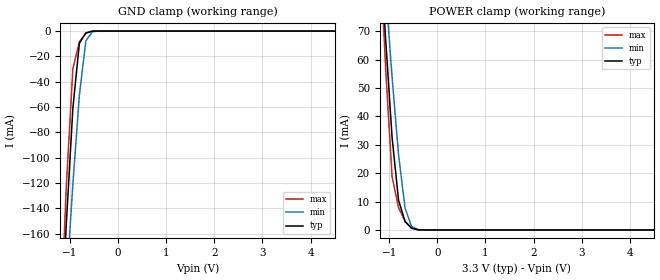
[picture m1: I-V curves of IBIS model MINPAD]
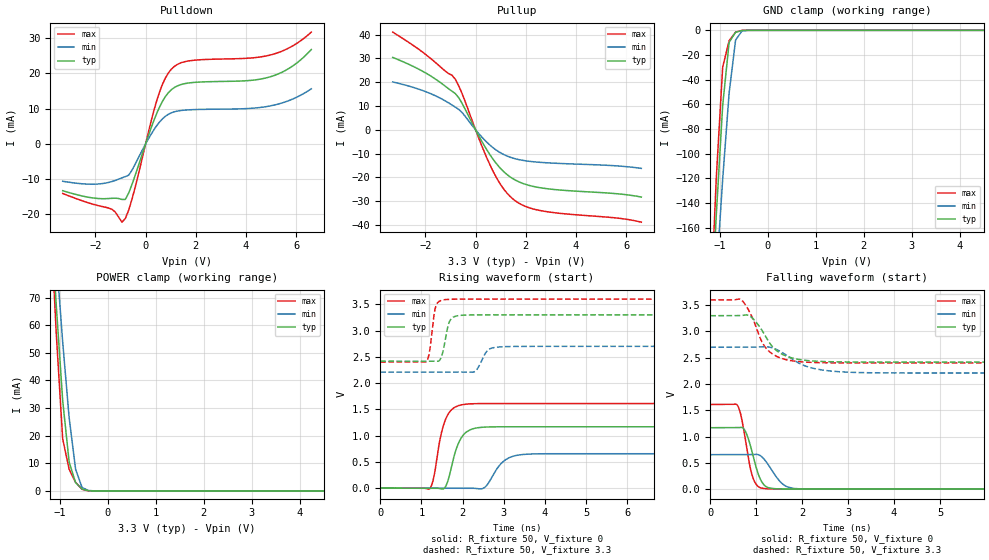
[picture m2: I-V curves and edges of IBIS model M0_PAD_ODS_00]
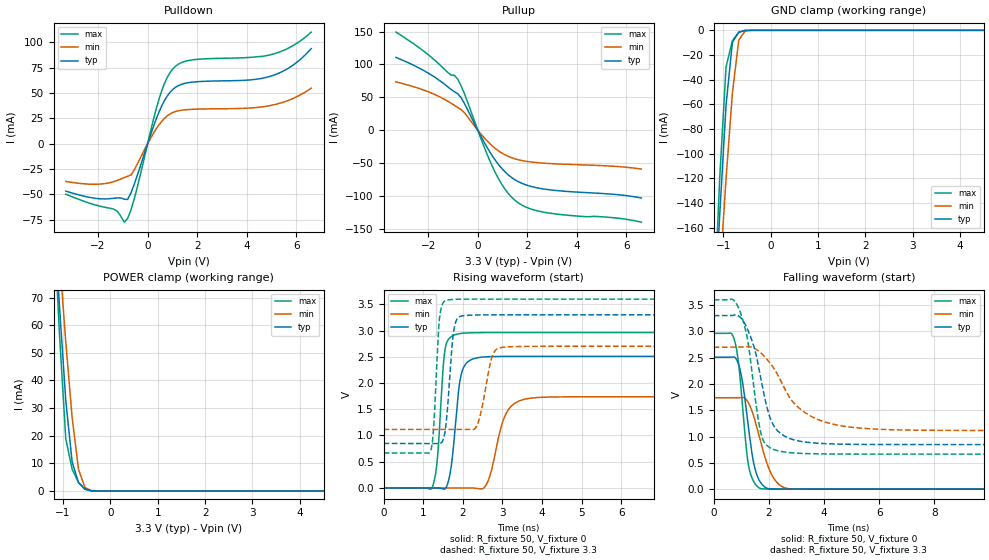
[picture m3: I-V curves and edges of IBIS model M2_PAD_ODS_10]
|   Microsemi Corporation
|   SmartFusion2 Automotive IBIS Model
[IBIS ver]   5.0
[File name]   as30208cc_33v_rev2p11.ibs
[File Rev]   2.11
[Date]   Wed Jul 17 2024
[Source] Simulated Models ONLY.
   All data is based on Spice simulation. All performed at Microsemi Corporation.
   Please refer to the Microsemi website for future updates at www.microsemi.com
[Notes]  Microsemi SmartFusion2 IBIS models for automotive operating conditions
   for DDRIO IO Banks IO Configurations ONLY. Models uses a software default
   fixed codes except for DDR3/SSTL15 which will always require calibrated
   codes.
   Automotive Temperature Grade 2 (t2) models cover a temperature range from
   -40C to 125C.
   Please refer to msio_auto_t2.ibs for MSIO IO Banks IO Configurations.
   Please refer to msiod_auto_t2.ibs for MSIOD IO Banks IO Configurations.
   The package parasitics of various package types are given.
   Uncomment the appropriate package or refer to the .pkg for specific
   per pin parasitic data.
   There are warnings related to non-monotonic and Increasing/Decreasing Current.
   They are expected on 20 Ohms and 30 Ohms I/O ODT models in DDR3/SSTL15.
[Disclaimer] This information is for board design considerations.
   Simulation based V/I curves contained in this model file are
   considered preliminary until verified against bench
   measurements. Maximum currents may vary from part to part but
   should not exceed maximum I/V curves provided in this model file.
[Copyright]  (c) 2015, Microsemi Corporation, All Rights Reserved.
| IBIS MODEL CHECKLIST
| Microsemi is dedicated to releasing quality IBIS models to customers.
| The following items have been
| verified for this IBIS model before release:
| 1)  Checked IBIS model by the golden parser ibischk5 [Complete]
| 2)  Ensured no errors reported by golden parser
|   for the IBIS model [Complete]
| 3)  Defined Vinl and Vinh for recievers [Complete]
| 4)  Defined Standard Load and Vmeas values for drivers [Complete]
| 5)  Defined overshoots for drivers and recievers [NA]
| 6)  Validated Ramp Values[Complete]
| 7)  Defined V-T Tables for all output drivers [Complete]
| 8)  Validated [Diff Pins] []
| 9)  Verified Package Parasitics [Complete]
| 10) Defined Standard Load Parameters and Specifications
|   for waveforms [Complete]
| 11) Defined and Validate Pin mappings [Complete]
| 12) Verified Ccomp Value []
| 13) Visually Inspected I-V Curves and V-T Tables  [Complete]
| 14) Presented Typ/Min/Max Values in the correct order for
|   all tables and parameters [Complete]
| 15) Simulated all output models with standard load and
|   switching through Vmeas [Complete]
| 16) Simulated all reciever models  [Complete]
| 17) Validated Models selectors. []
| 18) Visually inspected Spice and IBIS correlation for
|   a) Typical VT Curves [Complete]
|   b) Minimum VT Curves [Complete]
|   c) Maximum VT Curves [Complete]
| 19) Visually inspected Silicon and IBIS correlation
|   a) Typical IV Pull UP/ Pull Down Curves []
|   b) Minimum IV Pull UP/ Pull Down Curves []
|   c) Maximum IV Pull UP/ Pull Down Curves []
|   Component SmartFusion2
[Component]   SmartFusion2 W MRAM
[Manufacturer]   Avalanche Technology
[Package]
|  Design die-package: BGA
| variable   typ   min   max
R_pkg   0.72029   0.51528   1.0002
L_pkg   5.797e-9   4.155e-9   8.073e-9
C_pkg   1.116e-12   7.907e-13   1.753e-12
|Pin and Model info
[Pin]  signal_name  model_name   R_pin   L_pin   C_pin
L7   CS1#   MINPAD   0.4340		15.2000E-9		1.2600E-12
J8   CS2#   MINPAD   0.3800		13.5000E-9		1.0400E-12
K7   CLK1   MINPAD   0.4300		12.7000E-9		0.9790E-12
K6   CLK2   MINPAD   0.4480		14.6000E-9		1.1600E-12
M8   IO_0   MIOPAD   0.4010		12.4000E-9		1.2500E-12
M7   IO_1   MIOPAD   0.4050		14.2000E-9		1.1100E-12
L9   IO_2   MIOPAD   0.3780		11.8000E-9		1.2000E-12
M9   IO_3   MIOPAD   0.3700		11.8000E-9		1.2600E-12
M10   IO_4   MIOPAD   0.3710		11.1000E-9		1.1000E-12
N8   IO_5   MIOPAD   0.4050		13.8000E-9		1.1600E-12
N7   IO_6   MIOPAD   0.3830		15.2000E-9		1.0900E-12
N6   IO_7   MIOPAD   0.4480		16.4000E-9		1.0800E-12
J12   HTBSEL   MINPAD   0.1380		6.1700E-9		0.6060E-12
H12   HBP_2   MINPAD   0.1470		6.3900E-9		1.0000E-12
G11   HBP_1   MINPAD   0.1910		8.5000E-9		1.1500E-12
G10   HBP_0   MINPAD   0.2050		8.6800E-9		1.4200E-12
J9   RESET#   MINPAD   0.3410		14.1000E-9		1.6300E-12
J10   INT1#   MIOPAD   0.3080		12.5000E-9		1.2100E-12
K8   INT2#   MIOPAD   0.2120		10.3000E-9		0.8230E-12
M5   VSSIO   GND   NA   NA   NA
H6   VSSIO   GND   NA   NA   NA
L6   VSSIO   GND   NA   NA   NA
P8   VSSIO   GND   NA   NA   NA
H10   VSSIO   GND   NA   NA   NA
N10   VSSIO   GND   NA   NA   NA
P10   VSSIO   GND   NA   NA   NA
H11   VSSIO   GND   NA   NA   NA
N11   VSSIO   GND   NA   NA   NA
A1   VSS   GND   NA   NA   NA
B1   VSS   GND   NA   NA   NA
W1   VSS   GND   NA   NA   NA
Y1   VSS   GND   NA   NA   NA
A2   VSS   GND   NA   NA   NA
Y2   VSS   GND   NA   NA   NA
F3   VSS   GND   NA   NA   NA
G3   VSS   GND   NA   NA   NA
P3   VSS   GND   NA   NA   NA
R3   VSS   GND   NA   NA   NA
F4   VSS   GND   NA   NA   NA
H4   VSS   GND   NA   NA   NA
J4   VSS   GND   NA   NA   NA
L4   VSS   GND   NA   NA   NA
N4   VSS   GND   NA   NA   NA
R4   VSS   GND   NA   NA   NA
L5   VSS   GND   NA   NA   NA
N5   VSS   GND   NA   NA   NA
G6   VSS   GND   NA   NA   NA
P6   VSS   GND   NA   NA   NA
G8   VSS   GND   NA   NA   NA
H8   VSS   GND   NA   NA   NA
L10   VSS   GND   NA   NA   NA
L11   VSS   GND   NA   NA   NA
P11   VSS   GND   NA   NA   NA
F12   VSS   GND   NA   NA   NA
L12   VSS   GND   NA   NA   NA
N12   VSS   GND   NA   NA   NA
R12   VSS   GND   NA   NA   NA
F13   VSS   GND   NA   NA   NA
G13   VSS   GND   NA   NA   NA
P13   VSS   GND   NA   NA   NA
R13   VSS   GND   NA   NA   NA
A14   VSS   GND   NA   NA   NA
Y14   VSS   GND   NA   NA   NA
A15   VSS   GND   NA   NA   NA
B15   VSS   GND   NA   NA   NA
W15   VSS   GND   NA   NA   NA
Y15   VSS   GND   NA   NA   NA
G4   VCCIO   POWER   NA   NA   NA
P4   VCCIO   POWER   NA   NA   NA
G5   VCCIO   POWER   NA   NA   NA
J5   VCCIO   POWER   NA   NA   NA
P5   VCCIO   POWER   NA   NA   NA
M6   VCCIO   POWER   NA   NA   NA
H7   VCCIO   POWER   NA   NA   NA
H9   VCCIO   POWER   NA   NA   NA
N9   VCCIO   POWER   NA   NA   NA
J11   VCCIO   POWER   NA   NA   NA
M11   VCCIO   POWER   NA   NA   NA
G12   VCCIO   POWER   NA   NA   NA
P12   VCCIO   POWER   NA   NA   NA
K4   VCC   POWER   NA   NA   NA
M4   VCC   POWER   NA   NA   NA
K5   VCC   POWER   NA   NA   NA
G7   VCC   POWER   NA   NA   NA
P7   VCC   POWER   NA   NA   NA
G9   VCC   POWER   NA   NA   NA
K9   VCC   POWER   NA   NA   NA
P9   VCC   POWER   NA   NA   NA
K11   VCC   POWER   NA   NA   NA
K12   VCC   POWER   NA   NA   NA
M12   VCC   POWER   NA   NA   NA
| END PIN INFO
| IOPAD
[Model Selector] MIOPAD
| Model Description
M0_PAD_ODS_00   ODS_00
M1_PAD_ODS_01   ODS_01
M2_PAD_ODS_10   ODS_10
M3_PAD_ODS_11   ODS_11
| Models and submodels in the file (5): MINPAD (Input), M0_PAD_ODS_00 (I/O), M2_PAD_ODS_10 (I/O), M1_PAD_ODS_01 (I/O), M3_PAD_ODS_11 (I/O)
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[Model] MINPAD
Model_type Input
Enable   Active-High
Vinl  =  0.8
Vinh  =  2.2
| Capacitance  typ   min   max
C_comp   1.514821e-12   1.418868e-12   1.647023e-12
| Variables   typ   min   max
[GND Clamp Reference]   0   0   0
[POWER Clamp Reference]   3.3   2.7   3.6
[Pulldown Reference]   0   0   0
[Pullup Reference]   3.3   2.7   3.6
[Temperature Range]   25   125   -40
[Voltage Range]   3.3   2.7   3.6
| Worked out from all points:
|   GND clamp passes 1 mA (typ) near -0.62 V on its own axis
|   POWER clamp passes 1 mA (typ) near -0.56 V on its own axis
[GND Clamp]
| Voltage   I(typ)   I(min)   I(max)
-3.3V     -1.961A    -1.697A    -2.357A
-1.21V    -250.7mA   -283.7mA   -242.5mA
-1.076V   -150.6mA   -200.1mA   -120.6mA
-941.4mV  -60.83mA   -120.8mA   -29.75mA
-806.9mV  -9.646mA   -50.71mA   -8.435mA
-672.4mV  -1.585mA   -7.866mA   -1.457mA
-537.9mV  -71.75uA   -504.3uA   -18.73uA
-403.4mV  -593.9nA   -18.57uA   -37.22nA
6.6V      0A         0A         0A
[POWER Clamp]
| Voltage   I(typ)   I(min)   I(max)
-3.3V     772.3mA    673.3mA    930.5mA
-1.21V    105.9mA    117.6mA    104.6mA
-1.076V   67.34mA    85.06mA    57.16mA
-941.4mV  32.71mA    53.93mA    18.82mA
-806.9mV  10.48mA    26.53mA    7.848mA
-672.4mV  2.975mA    7.856mA    3.108mA
-537.9mV  710.9uA    1.248mA    573.1uA
-403.4mV  60.69uA    160.8uA    9.187uA
-269mV    142.4nA    6.118uA    23.26nA
6.6V      0A         0A         0A
[Model] M0_PAD_ODS_00
Model_type I/O
Enable   Active-High
Vinl  =  0.8
Vinh  =  2.2
Vmeas =  1.65
Cref  =  30e-12
| Capacitance  typ   min   max
C_comp   1.518749e-12   1.424706e-12   1.652746e-12
| Variables   typ   min   max
[GND Clamp Reference]   0   0   0
[POWER Clamp Reference]   3.3   2.7   3.6
[Pulldown Reference]   0   0   0
[Pullup Reference]   3.3   2.7   3.6
[Temperature Range]   25   125   -40
[Voltage Range]   3.3   2.7   3.6
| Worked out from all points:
|   slope of the pulldown table from 0 to 0.495 V, typ, clamps not added: 52.1 ohm
|   slope of the pullup table from 0 to 0.495 V, typ, clamps not added: 53.8 ohm
|   GND clamp passes 1 mA (typ) near -0.62 V on its own axis
|   POWER clamp passes 1 mA (typ) near -0.56 V on its own axis
|   falling waveform, R_fixture 50, V_fixture 0: 20-80 % time 230ps typ, 320ps min, 198ps max; typ from 1.17 V to 0 V
|   falling waveform, R_fixture 50, V_fixture 3.3: 20-80 % time 464ps typ, 644ps min, 396ps max; typ from 3.3 V to 2.42 V
|   rising waveform, R_fixture 50, V_fixture 0: 20-80 % time 273ps typ, 362ps min, 248ps max; typ from 0 V to 1.17 V
|   rising waveform, R_fixture 50, V_fixture 3.3: 20-80 % time 138ps typ, 198ps min, 114ps max; typ from 2.42 V to 3.3 V
[GND Clamp]
| Voltage   I(typ)   I(min)   I(max)
-3.3V     -1.961A    -1.697A    -2.357A
-1.21V    -250.7mA   -283.7mA   -242.5mA
-1.076V   -150.6mA   -200.1mA   -120.7mA
-941.4mV  -60.83mA   -120.8mA   -29.76mA
-806.9mV  -9.649mA   -50.71mA   -8.442mA
-672.4mV  -1.587mA   -7.866mA   -1.46mA
-537.9mV  -71.93uA   -504.3uA   -18.83uA
-403.4mV  -595.6nA   -18.58uA   -37.45nA
6.6V      0A         0A         0A
[POWER Clamp]
| Voltage   I(typ)   I(min)   I(max)
-3.3V     772.3mA    673.3mA    930.5mA
-1.21V    105.9mA    117.6mA    104.6mA
-1.076V   67.34mA    85.06mA    57.16mA
-941.4mV  32.71mA    53.93mA    18.82mA
-806.9mV  10.48mA    26.53mA    7.848mA
-672.4mV  2.975mA    7.856mA    3.108mA
-537.9mV  710.9uA    1.248mA    573.1uA
-403.4mV  60.69uA    160.8uA    9.187uA
-269mV    142.4nA    6.118uA    23.26nA
6.6V      0A         0A         0A
[Pulldown]
| Voltage   I(typ)   I(min)   I(max)
-3.3V     -13.26mA   -10.58mA   -14.05mA
-1.345V   -15.42mA   -10.67mA   -18.51mA
-941.4mV  -15.74mA   -9.611mA   -22.19mA
-806.9mV  -15.73mA   -9.263mA   -21.14mA
-537.9mV  -11.42mA   -7.417mA   -15.59mA
455.2mV   8.881mA    5.308mA    12.55mA
682.8mV   12.23mA    7.205mA    17.1mA
1.024V    15.38mA    8.837mA    21.2mA
1.821V    17.39mA    9.724mA    23.68mA
4.914V    18.96mA    10.73mA    25.16mA
5.783V    21.77mA    12.53mA    27.53mA
6.6V      26.8mA     15.66mA    31.75mA
[Pullup]
| Voltage   I(typ)   I(min)   I(max)
-3.3V     30.44mA    20.14mA    41.1mA
-1.883V   23.26mA    15.61mA    30.81mA
-806.9mV  15.23mA    9.539mA    21.27mA
-537.9mV  11.14mA    7.294mA    15.26mA
227.6mV   -4.448mA   -2.796mA   -6.209mA
682.8mV   -12.17mA   -7.42mA    -17.15mA
1.138V    -17.78mA   -10.49mA   -25.16mA
1.593V    -21.21mA   -12.21mA   -29.96mA
2.048V    -23.14mA   -13.13mA   -32.47mA
2.731V    -24.61mA   -13.8mA    -34.27mA
5.659V    -26.92mA   -15.2mA    -37.16mA
6.6V      -28.29mA   -16.23mA   -38.86mA
[Ramp]
dV/dt_r   0.701574/0.273396n  0.393696/0.362182n  0.967082/0.24767n
dV/dt_f   0.529393/0.463707n  0.294233/0.644316n  0.719379/0.396117n
R_load = 50
[Falling Waveform]
R_fixture = 50
V_fixture = 0
V_fixture_min = 0
V_fixture_max = 0
| Time   V(typ)   V(min)   V(max)
0s        1.169V     656.2mV    1.612V
592.6ps   1.17V      656.6mV    1.594V
662.7ps   1.175V     656.6mV    1.423V
757.8ps   1.11V      656.7mV    979.6mV
920.8ps   673.8mV    658.3mV    236.4mV
1.068ns   233.8mV    649.1mV    35.66mV
1.221ns   45.34mV    516.2mV    8.708mV
1.592ns   3.21mV     87.01mV    1.102mV
2.018ns   581.9uV    4.7mV      706uV
21.88ns   211nV      -2.279uV   3.818uV
[Falling Waveform]
R_fixture = 50
V_fixture = 3.3
V_fixture_min = 2.7
V_fixture_max = 3.6
| Time   V(typ)   V(min)   V(max)
0s        3.3V       2.7V       3.6V
662.6ps   3.302V     2.701V     3.609V
894.9ps   3.273V     2.701V     3.302V
1.117ns   3.036V     2.709V     2.815V
1.233ns   2.866V     2.709V     2.664V
1.51ns    2.594V     2.628V     2.502V
2.006ns   2.457V     2.366V     2.42V
2.5ns     2.427V     2.259V     2.405V
3.502ns   2.418V     2.214V     2.401V
21.88ns   2.418V     2.21V      2.401V
[Rising Waveform]
R_fixture = 50
V_fixture = 0
V_fixture_min = 0
V_fixture_max = 0
| Time   V(typ)   V(min)   V(max)
0s        11.89nV    88.47nV    -73.19nV
1.207ns   -862.4uV   -520.5uV   -4.427mV
1.285ns   -918.3uV   -554.2uV   157.9mV
1.593ns   39.36mV    -686.9uV   1.324V
1.858ns   773.7mV    -801.1uV   1.558V
2.069ns   1.055V     -892.4uV   1.599V
2.519ns   1.162V     5.17mV     1.611V
2.991ns   1.169V     510.2mV    1.611V
3.605ns   1.169V     648.6mV    1.611V
21.88ns   1.169V     656.2mV    1.612V
[Rising Waveform]
R_fixture = 50
V_fixture = 3.3
V_fixture_min = 2.7
V_fixture_max = 3.6
| Time   V(typ)   V(min)   V(max)
0s        2.418V     2.21V      2.401V
1.115ns   2.419V     2.21V      2.406V
1.19ns    2.419V     2.21V      2.571V
1.354ns   2.418V     2.21V      3.473V
1.494ns   2.522V     2.21V      3.578V
1.647ns   3.091V     2.21V      3.594V
2.284ns   3.299V     2.216V     3.599V
2.637ns   3.299V     2.641V     3.599V
3.102ns   3.299V     2.696V     3.599V
21.88ns   3.3V       2.7V       3.6V
[Model] M2_PAD_ODS_10
Model_type I/O
Enable   Active-High
Vinl  =  0.8
Vinh  =  2.2
Vmeas =  1.65
Cref  =  30e-12
| Capacitance  typ   min   max
C_comp   1.518749e-12   1.424706e-12   1.652746e-12
| Variables   typ   min   max
[GND Clamp Reference]   0   0   0
[POWER Clamp Reference]   3.3   2.7   3.6
[Pulldown Reference]   0   0   0
[Pullup Reference]   3.3   2.7   3.6
[Temperature Range]   25   125   -40
[Voltage Range]   3.3   2.7   3.6
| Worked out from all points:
|   slope of the pulldown table from 0 to 0.495 V, typ, clamps not added: 14.9 ohm
|   slope of the pullup table from 0 to 0.495 V, typ, clamps not added: 14.7 ohm
|   GND clamp passes 1 mA (typ) near -0.62 V on its own axis
|   POWER clamp passes 1 mA (typ) near -0.56 V on its own axis
|   falling waveform, R_fixture 50, V_fixture 0: 20-80 % time 394ps typ, 590ps min, 315ps max; typ from 2.51 V to 0 V
|   falling waveform, R_fixture 50, V_fixture 3.3: 20-80 % time 660ps typ, 1.32ns min, 479ps max; typ from 3.3 V to 0.848 V
|   rising waveform, R_fixture 50, V_fixture 0: 20-80 % time 197ps typ, 348ps min, 149ps max; typ from 0 V to 2.51 V
|   rising waveform, R_fixture 50, V_fixture 3.3: 20-80 % time 147ps typ, 240ps min, 115ps max; typ from 0.848 V to 3.3 V
[GND Clamp]
| Voltage   I(typ)   I(min)   I(max)
-3.3V     -1.961A    -1.697A    -2.357A
-1.21V    -250.7mA   -283.7mA   -242.5mA
-1.076V   -150.6mA   -200.1mA   -120.7mA
-941.4mV  -60.83mA   -120.8mA   -29.76mA
-806.9mV  -9.649mA   -50.71mA   -8.442mA
-672.4mV  -1.587mA   -7.866mA   -1.46mA
-537.9mV  -71.93uA   -504.3uA   -18.83uA
-403.4mV  -595.6nA   -18.58uA   -37.45nA
6.6V      0A         0A         0A
[POWER Clamp]
| Voltage   I(typ)   I(min)   I(max)
-3.3V     772.3mA    673.3mA    930.5mA
-1.21V    105.9mA    117.6mA    104.6mA
-1.076V   67.34mA    85.06mA    57.16mA
-941.4mV  32.71mA    53.93mA    18.82mA
-806.9mV  10.48mA    26.53mA    7.848mA
-672.4mV  2.975mA    7.856mA    3.108mA
-537.9mV  710.9uA    1.248mA    573.1uA
-403.4mV  60.69uA    160.8uA    9.187uA
-269mV    142.4nA    6.118uA    23.26nA
6.6V      0A         0A         0A
[Pulldown]
| Voltage   I(typ)   I(min)   I(max)
-3.3V     -46.77mA   -37.16mA   -49.83mA
-1.345V   -53.76mA   -37.21mA   -64.77mA
-941.4mV  -54.71mA   -33.33mA   -77.43mA
-806.9mV  -55.02mA   -32.17mA   -73.73mA
-537.9mV  -39.9mA    -25.92mA   -54.28mA
455.2mV   31.02mA    18.55mA    43.7mA
682.8mV   42.73mA    25.18mA    59.65mA
1.024V    53.77mA    30.89mA    74.07mA
1.821V    60.81mA    33.99mA    82.81mA
4.914V    66.31mA    37.51mA    87.55mA
5.783V    76.16mA    43.8mA     95.68mA
6.6V      93.82mA    54.81mA    110.2mA
[Pullup]
| Voltage   I(typ)   I(min)   I(max)
-3.3V     110.8mA    73.4mA     149.4mA
-1.883V   84.27mA    56.72mA    111.4mA
-806.9mV  55.48mA    34.56mA    77.7mA
-537.9mV  40.72mA    26.67mA    55.72mA
227.6mV   -16.26mA   -10.22mA   -22.67mA
682.8mV   -44.48mA   -27.12mA   -62.65mA
1.138V    -65.01mA   -38.35mA   -91.97mA
1.593V    -77.56mA   -44.65mA   -109.6mA
2.162V    -85.85mA   -48.54mA   -120.3mA
2.845V    -90.61mA   -50.73mA   -126.1mA
5.534V    -97.91mA   -55.15mA   -133.7mA
6.6V      -103.4mA   -59.29mA   -140.2mA
[Ramp]
dV/dt_r   1.50494/0.197293n  1.04234/0.347547n  1.77705/0.14905n
dV/dt_f   1.47118/0.66022n  0.951015/1.316n  1.76015/0.479444n
R_load = 50
[Falling Waveform]
R_fixture = 50
V_fixture = 0
V_fixture_min = 0
V_fixture_max = 0
| Time   V(typ)   V(min)   V(max)
0s        2.508V     1.737V     2.962V
759.6ps   2.508V     1.738V     2.821V
890.4ps   2.387V     1.738V     2.436V
999.8ps   2.164V     1.741V     1.857V
1.254ns   1.197V     1.646V     471.7mV
1.462ns   460.6mV    1.364V     132.2mV
1.72ns    111.8mV    859.7mV    7.736mV
2.149ns   3.807mV    230.1mV    1.501mV
2.718ns   1.059mV    9.353mV    845.9uV
21.88ns   537.2nV    325.5nV    -804nV
[Falling Waveform]
R_fixture = 50
V_fixture = 3.3
V_fixture_min = 2.7
V_fixture_max = 3.6
| Time   V(typ)   V(min)   V(max)
0s        3.3V       2.7V       3.6V
659.1ps   3.3V       2.7V       3.614V
907.4ps   3.292V     2.701V     3.438V
1.244ns   3.017V     2.711V     2.79V
1.71ns    2.099V     2.591V     1.067V
2ns       1.425V     2.426V     802.7mV
2.308ns   1.117V     2.186V     732.6mV
3.226ns   902.4mV    1.487V     679.2mV
4.9ns     853.7mV    1.183V     667.3mV
21.88ns   848mV      1.115V     666.4mV
[Rising Waveform]
R_fixture = 50
V_fixture = 0
V_fixture_min = 0
V_fixture_max = 0
| Time   V(typ)   V(min)   V(max)
0s        5.777nV    44.9nV     -42.68nV
1.217ns   886.5uV    -289.8uV   -4.263mV
1.357ns   1.052mV    -323.2uV   556.4mV
1.551ns   -16.19mV   -369.6uV   2.647V
1.711ns   437.6mV    -407.7uV   2.887V
1.916ns   1.993V     -456.6uV   2.942V
2.553ns   2.498V     17.69mV    2.961V
3.099ns   2.508V     1.428V     2.962V
3.73ns    2.508V     1.712V     2.962V
21.88ns   2.508V     1.737V     2.962V
[Rising Waveform]
R_fixture = 50
V_fixture = 3.3
V_fixture_min = 2.7
V_fixture_max = 3.6
| Time   V(typ)   V(min)   V(max)
0s        848mV      1.115V     666.4mV
1.189ns   847.3mV    1.116V     714.5mV
1.41ns    844.8mV    1.116V     3.235V
1.604ns   1.442V     1.116V     3.581V
1.773ns   3.011V     1.116V     3.594V
2.021ns   3.283V     1.116V     3.599V
2.351ns   3.297V     1.183V     3.599V
2.742ns   3.299V     2.508V     3.599V
3.026ns   3.299V     2.682V     3.599V
21.88ns   3.3V       2.7V       3.6V
